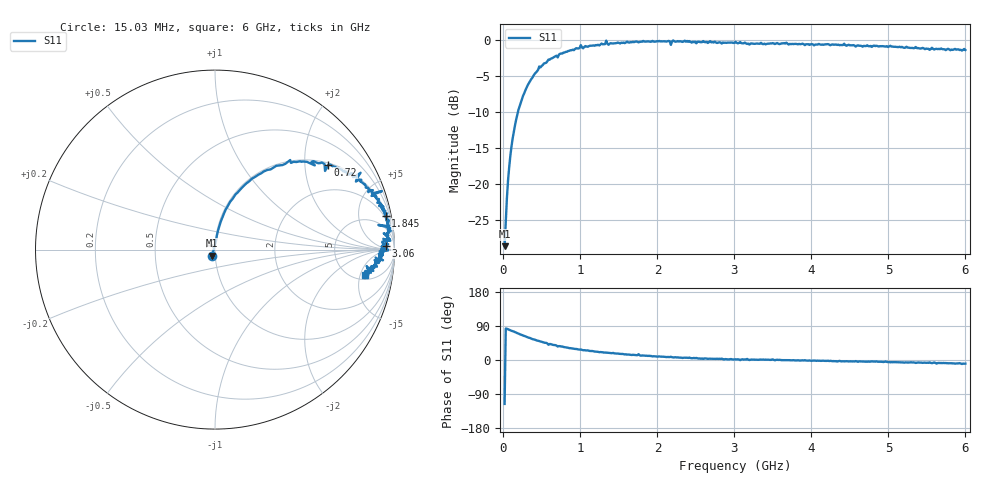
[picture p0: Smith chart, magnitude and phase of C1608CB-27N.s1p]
!	Network	Analyzer	HP8753E.07.74:	Oct	30	2002	Serial	No.	JP38451487
!	Hewlett-Packard
!	7	Sep	2009	9:41:10
!	Frequency	S11
#	HZ	S	RI	R	50
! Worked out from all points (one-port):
!   400 points, 15.03 MHz to 6 GHz, reference 50 ohm
!   lowest |S11| = -28.7 dB at 15.03 MHz (marker M1), VSWR 1.08, Z = 48.3 - j3.21 ohm
!   |S11| at or under -10 dB: start of sweep to 189.3 MHz
!   S11 on the Smith chart (normalised r, x): 15.03 MHz: 0.97, -0.06; 720 MHz: 1.06, +2.63; 1.845 GHz: 2, +10; 3.06 GHz: 33, +15; 6 GHz: 6.01, -6.03
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1.502992e7  -0.0161 -0.0332
4.502978e7  0.0105 0.0791
7.502962e7  0.0239 0.129
1.200294e8  0.0501 0.201
1.95029e8  0.113 0.306
4.650277e8  0.419 0.499
7.200264e8  0.631 0.471
7.650262e8  0.652 0.466
1.005025e9  0.811 0.428
1.035025e9  0.785 0.379
1.320023e9  0.878 0.314
1.335023e9  0.93 0.326
1.365023e9  0.872 0.299
1.515022e9  0.904 0.261
1.740021e9  0.944 0.213
1.755021e9  0.923 0.256
1.785021e9  0.95 0.19
1.845021e9  0.951 0.187
2.145019e9  0.971 0.134
2.175019e9  0.91 0.137
2.205019e9  0.981 0.116
2.265019e9  0.971 0.116
3.015015e9  0.965 0.0301
3.060015e9  0.951 0.022
3.765011e9  0.932 -0.00717
4.515007e9  0.913 -0.0558
5.265004e9  0.875 -0.101
6e9  0.836 -0.141
